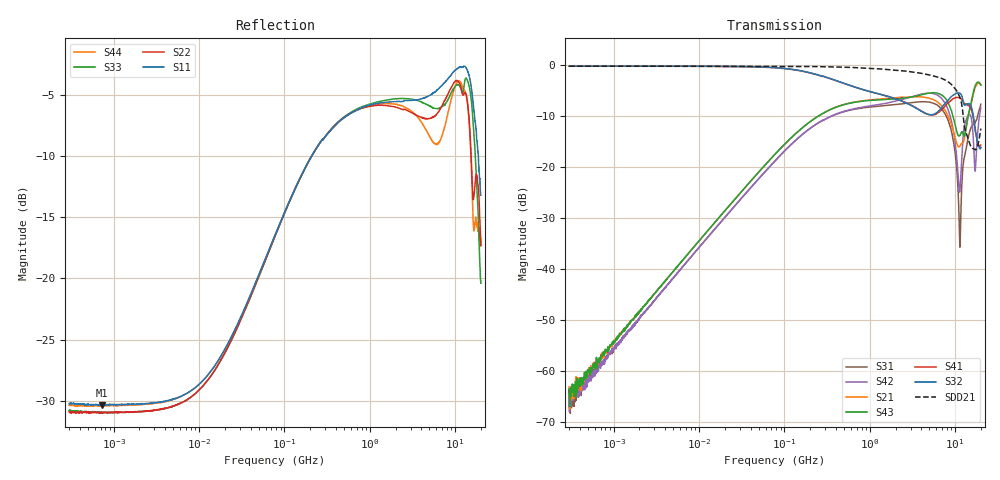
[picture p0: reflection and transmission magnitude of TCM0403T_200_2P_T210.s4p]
! S-Parameter Data Generated by TDK Corporation
! Copyright(C) 2024 TDK Corporation.
! All Rights Reserved.
! TDK P/N: TCM0403T-200-2P-T210 (Signal Line Common Mode Choke/Filter)
! Property: -
! Size(LxWxT): 0.45x0.3x0.23mm
! Model Type: s2p (Touchstone File Format Version 1.0)
! Frequency: DC=Yes Start=0.3MHz Stop=20000MHz 1602points Log-sweep
! Model Generated on May 28, 2024
! Terms and conditions regarding TDK Simulation Models:
! 1)This simulation model is being provided solely for informational
!  purposes. Please refer to the specifications of the products in
!  terms of detailed characteristics of such products.
! 2)In no event shall TDK Corporation of any of its subsidiaries be
!  liable for any loss or damage arising, directly or indirectly,
!  from any information contained in this simulation model, including,
!  but not limited to loss or damages arising from any inaccuracies,
!  omissions or errors in connection with such information.
! 3)Any and all copyrights on this simulation model are owned by
!  TDK Corporation.  Duplication or redistribution of this simulation
!  model without prior written permission from TDK Corporation
!  is prohibited.
! 4)This simulation model is subject to any modification or change
!  without any prior notice.
! 5)Neither TDK Corporation nor any of its subsidiaries shall make any
!  warranty, express or implied, including but not limited to the
!  correctness, implied warranties of merchantability and fitness for
!  a particular purpose with respect to this simulation models.
! 6)The use of this simulation model shall be deemed to have consented
!  to the terms and conditions hereof.
! Port Assignments:
!  1 ---@@@--- 4
!  2 ---@@@--- 3
! Applicable Conditions:
!  Temperature = 25 degC
!  DC Bias Current = 0 A
!  Small Signal Operation
# Hz S MA R 50
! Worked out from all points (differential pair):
!   1601 points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, 300 kHz to 20 GHz, reference 50 ohm
!   strongest paths, dB at 300 kHz, 4.882 MHz, 77.46 MHz, 1.261 GHz, 20 GHz:
!     S32: -0.3, -0.3, -0.5, -5.7, -16.2
!     S41: -0.3, -0.3, -0.6, -5.7, -15.7
!     S43: -64.8, -40.7, -17.5, -6.8, -4.0
!     S21: -63.2, -40.7, -17.5, -6.7, -3.9
!     S42: -64.3, -42.0, -18.8, -7.8, -8.4
!     S31: -63.8, -42.0, -18.8, -8.1, -7.7
!   taken as a pair (ports 2,1 in; 3,4 out), SDD21 dB: -0.3, -0.3, -0.3, -0.8, -12.5
!   lowest |S11| = -30.4 dB at 726.9 kHz (marker M1), VSWR 1.06, Z = 53.1 + j0.0602 ohm
!   |S11| at or under -10 dB: start of sweep to 208.6 MHz; 18.69 GHz to end of sweep
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300000  0.03078 -1.8  0.0006965 86.2  0.0005066 -97.1  0.9688 -0.0
        0.0006938 89.8  0.02851 0.4  0.9715 -0.1  0.0005685 -79.6
        0.0006484 -99.2  0.9711 -0.0  0.0289 -0.4  0.0006549 91.1
        0.97 -0.1  0.0006126 -91.9  0.0005722 85.2  0.03037 -0.4
726922  0.03037 1.1  0.001332 89.4  0.001158 -93.0  0.9695 -0.1
        0.001429 90.0  0.02842 2.3  0.9715 -0.1  0.001186 -89.8
        0.001174 -86.9  0.9716 -0.1  0.02846 2.0  0.001321 91.3
        0.9698 -0.1  0.001181 -90.6  0.001398 89.2  0.03037 2.2
2.075857e8  0.3154 46.7  0.284 50.2  0.244 -136.2  0.8272 -19.8
            0.284 50.2  0.3151 46.7  0.831 -19.9  0.2441 -137.1
            0.2439 -136.2  0.8309 -19.9  0.3156 47.4  0.2839 50.3
            0.8269 -19.8  0.2443 -137.1  0.2839 50.3  0.3154 45.9
1.373372e9  0.5217 8.7  0.4639 7.8  0.3957 148.7  0.5103 -44.8
            0.4638 7.9  0.5099 4.0  0.5109 -44.8  0.4139 142.9
            0.3959 148.9  0.5103 -44.9  0.5297 7.3  0.4565 9.1
            0.5109 -44.6  0.4133 142.8  0.4565 9.1  0.5166 2.7
5.99646e9  0.5828 -8.3  0.4411 -26.7  0.4068 28.3  0.3314 176.7
           0.441 -26.7  0.4657 -12.2  0.3379 170.4  0.5129 19.9
           0.4089 28.1  0.3374 170.8  0.494 -19.1  0.5323 -18.7
           0.331 176.5  0.5118 20.3  0.5322 -18.6  0.353 -15.6
1.134441e10  0.7294 -39.5  0.1599 -6.5  0.01633 -157.1  0.4739 50.7
             0.1599 -6.4  0.6208 -51.6  0.5307 43.4  0.05921 17.6
             0.01628 -156.6  0.5284 43.7  0.6063 -46.3  0.2031 -17.9
             0.4738 51.3  0.05795 18.0  0.2029 -17.7  0.6358 -47.0
2e10  0.2187 -92.6  0.6415 -32.3  0.4119 33.6  0.17 37.5
      0.6417 -32.2  0.1358 -103.0  0.1551 32.7  0.3802 30.6
      0.4117 33.9  0.155 33.5  0.09566 -92.4  0.633 -43.7
      0.1636 37.5  0.3808 30.1  0.6327 -43.4  0.1365 -72.3
